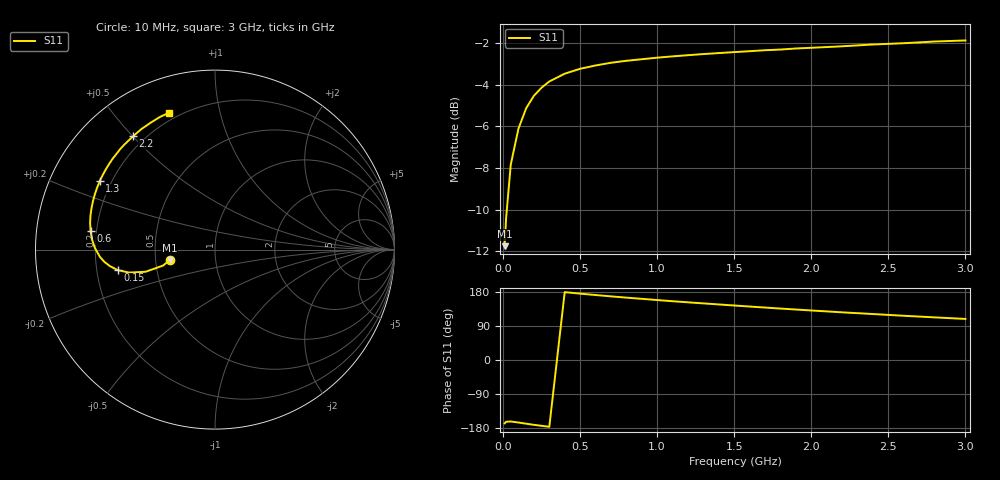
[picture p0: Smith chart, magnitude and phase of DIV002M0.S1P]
! SIEMENS Small Signal Semiconductors
! BAV99
! Silicon Switching Diode in SOT23
! IF = 2 mA
! S-Parameters:  May  1995
# GHz  S  MA  R  50
!  f  S11
! GHz  MAG  ANG
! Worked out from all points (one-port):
!   30 points, 10 MHz to 3 GHz, reference 50 ohm
!   lowest |S11| = -11.7 dB at 10 MHz (marker M1), VSWR 1.70, Z = 29.7 - j3.68 ohm
!   |S11| at or under -10 dB: start of sweep to 24.43 MHz
!   S11 on the Smith chart (normalised r, x): 10 MHz: 0.59, -0.07; 150 MHz: 0.29, -0.10; 600 MHz: 0.18, +0.07; 1.3 GHz: 0.16, +0.27; 2.2 GHz: 0.16, +0.50; 3 GHz: 0.16, +0.71
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0.01  0.2587 -167.1
0.02  0.3028 -162.9
0.05  0.4058 -162.3
0.1  0.495 -165.0
0.15  0.5538 -168.1
0.2  0.5931 -171.1
0.25  0.6203 -173.7
0.3  0.6419 -176.3
0.4  0.67 179.1
0.5  0.6884 175.1
0.6  0.7011 171.5
0.7  0.7116 167.9
0.8  0.7195 164.6
0.9  0.7257 161.4
1  0.7319 158.2
1.1  0.7372 155.1
1.2  0.742 152.2
1.3  0.7467 149.4
1.4  0.7508 146.6
1.6  0.7586 141.1
1.7  0.7627 138.4
1.9  0.7701 133.2
2  0.773 130.7
2.2  0.7793 125.8
2.4  0.7871 121.3
2.6  0.7928 116.7
2.8  0.8002 112.5
3  0.8049 108.4
